(* Logix 5000 Rung export; software revision 17.00 *)

TYPE AENWG_CIP :   // Total Number of Current CIP Connections
STRUCT
   Opens : DINT;   // Total number of CIP connection Open Requests
   Closes : DINT;   // Total Number of CIP Connection Close Requests
   TimeOuts : DINT;   // Total Number of CIP Connection TimeOuts
END_STRUCT
END_TYPE

TYPE AENWG_PacketsRxSuccess :
STRUCT
   TotalCount : DINT;   // Total number of "good" received packets
   AvgPerSecond : DINT;   // Average "good" received packets per second
END_STRUCT
END_TYPE

TYPE AENWG_PacketsTxRetries :
STRUCT
   TotalCount : DINT;   // Total transmit packet retries
   AvgPerSecond : DINT;   // Average transmit packet retries per second
END_STRUCT
END_TYPE

TYPE AENWG_PacketsTxSuccess :
STRUCT
   TotalCount : DINT;   // Total "good" transmitted packets
   AvgPerSecond : DINT;   // Average "good" transmitted packets per second
END_STRUCT
END_TYPE

TYPE AENWG_PacketsTxFailures :
STRUCT
   TotalCount : DINT;   // Total number of failed transmitted packets
   AvgPerSecond : DINT;   // Average failed packets per second
END_STRUCT
END_TYPE

TYPE AENWG_RadioLinkTime :
STRUCT
   Days : INT;   // Number of days the radio has been linked to a parent
   Hours : INT;   // Number of hours the radio has been linked to a parent
   Minutes : INT;   // Number of minutes the radio has been linked to a parent
   Seconds : INT;   // Number of seconds the radio has been linked to a parent
END_STRUCT
END_TYPE

TYPE AENWG_DIAGNOSTICS :
STRUCT
   Control : AENWG_CONTROL;
   HMI : AENWG_HMI;
END_STRUCT
END_TYPE

TYPE AENWG_HMI :
STRUCT
   Face_Plate_Nav : DINT;   // Used by the HMI for display navigation
   RadioFirmware : DINT;   // Current radio firmware revision
   Module_Comm_Status : INT;
   ParentDataRate : INT;   // The data rate at which the parent is transmitting data *IN Mbps
   RSSI : INT;   // Current receive signal strength
   SignalToNoise : INT;   // Current noise level
   LinkTime : AENWG_RadioLinkTime;   // Total time the radio has been linked to a master
   ParentMACaddress : AENWG_ParentMACAddress;   // The MAC address of the linked parent
   TxPackets_Success : AENWG_PacketsTxSuccess;   // Total and average "good" packets
   TxPackets_Fail : AENWG_PacketsTxFailures;   // Total and average failed packets
   TxPackets_Retries : AENWG_PacketsTxRetries;   // Total and average retries
   RxPackets_Success : AENWG_PacketsRxSuccess;   // Total and average received packets
   IPInformation : AENWG_IPData;   // ILX34 TCP information
   CIP : AENWG_CIP;   // ILX34 CIP Connection Data
END_STRUCT
END_TYPE

TYPE AENWG_ParentMACAddress :
STRUCT
   Octet1 : SINT;   // Octet1 of the parent's MAC address
   Octet2 : SINT;   // Octet2 of the parent's MAC address
   Octet3 : SINT;   // Octet3 of the parent's MAC address
   Octet4 : SINT;   // Octet4 of the parent's MAC address
   Octet5 : SINT;   // Octet5 of the parent's MAC address
   Octet6 : SINT;   // Octet6 of the parent's MAC address
END_STRUCT
END_TYPE

TYPE AENWG_IPData :   // contains the IP information related to the ILX34.
STRUCT
   IPAddress : INT[4];
   NetworkSubMask : INT[4];
   GatewayAddress : INT[4];
   DNSServer : INT[4];
   DNSServer2 : INT[4];
   IP_Msg_Trigger : DINT;
END_STRUCT
END_TYPE

TYPE AENWG_CONTROL :
STRUCT
   ConMsgData : INT[12];   // Array that stores temporary connection data from the ILX34
   RadioMsgData : INT[36];   // Array that stores the temporary data from the ILX34
   IPMsgData : DINT[10];   // Array that stores temporary data for the IP information
   PollRate : DINT;   // Poll rate for retrieving radio diagnostic data *IN SECONDS
   RadioPollTimer : TIMER;   // Interval at which to get diagnostics from the ILX34 (should not be faster than every 3 sec)
END_STRUCT
END_TYPE

ADD_ON_INSTRUCTION ILX34AENWG_Advanced   (* revision 1.0, vendor ProSoft Technology, ExecutePrescan *)
// This is the Advanced Add On Instruction that provides the ability to get diagnostic information from an ILX34AENWG.
VAR_IN_OUT
   ILX34_Diag_msg : MESSAGE; {required}
   WirelessAENWG_Diags : AENWG_DIAGNOSTICS; {required}
   ILX34_IP_Info_msg : MESSAGE; {required}
   ILX34_Con_Diag_msg : MESSAGE; {required}
END_VAR
VAR
   Move_IP_Data : BOOL;
   IP_Domain_Name_Size : DINT;
   Move_Wireless_Diag : BOOL;
END_VAR

ROUTINE Logic   (* ladder *)
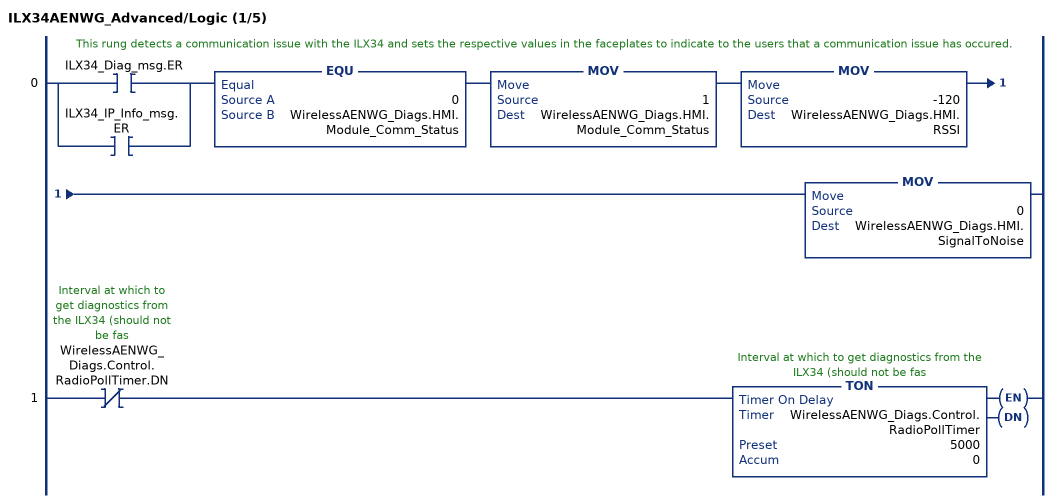
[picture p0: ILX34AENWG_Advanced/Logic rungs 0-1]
   // This rung detects a communication issue with the ILX34 and sets the respective values in the faceplates to indicate to the users that a communication issue has occured.
   0: [XIC(ILX34_Diag_msg.ER) ,XIC(ILX34_IP_Info_msg.ER) ]EQU(0,WirelessAENWG_Diags.HMI.Module_Comm_Status)MOV(1,WirelessAENWG_Diags.HMI.Module_Comm_Status)MOV(-120,WirelessAENWG_Diags.HMI.RSSI)MOV(0,WirelessAENWG_Diags.HMI.SignalToNoise);
   1: XIO(WirelessAENWG_Diags.Control.RadioPollTimer.DN)TON(WirelessAENWG_Diags.Control.RadioPollTimer,5000,0);
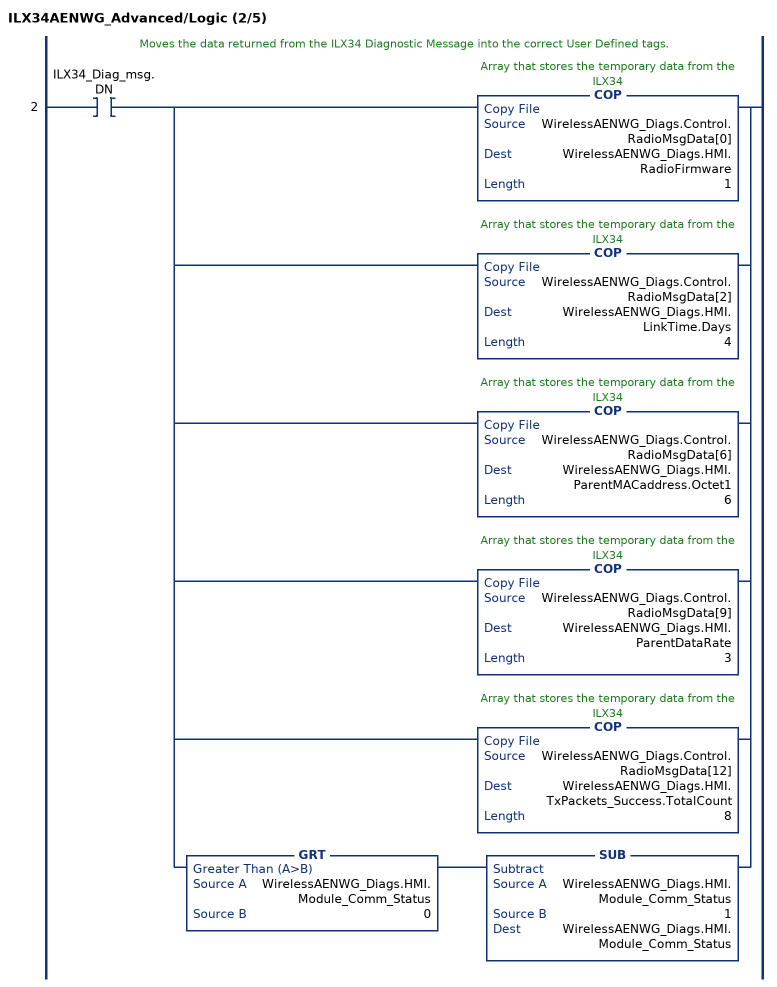
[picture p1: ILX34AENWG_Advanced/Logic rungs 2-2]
   // Moves the data returned from the ILX34 Diagnostic Message into the correct User Defined tags.
   2: XIC(ILX34_Diag_msg.DN)[COP(WirelessAENWG_Diags.Control.RadioMsgData[0],WirelessAENWG_Diags.HMI.RadioFirmware,1) ,COP(WirelessAENWG_Diags.Control.RadioMsgData[2],WirelessAENWG_Diags.HMI.LinkTime.Days,4) ,COP(WirelessAENWG_Diags.Control.RadioMsgData[6],WirelessAENWG_Diags.HMI.ParentMACaddress.Octet1,6) ,COP(WirelessAENWG_Diags.Control.RadioMsgData[9],WirelessAENWG_Diags.HMI.ParentDataRate,3) ,COP(WirelessAENWG_Diags.Control.RadioMsgData[12],WirelessAENWG_Diags.HMI.TxPackets_Success.TotalCount,8) ,GRT(WirelessAENWG_Diags.HMI.Module_Comm_Status,0) SUB(WirelessAENWG_Diags.HMI.Module_Comm_Status,1,WirelessAENWG_Diags.HMI.Module_Comm_Status) ];
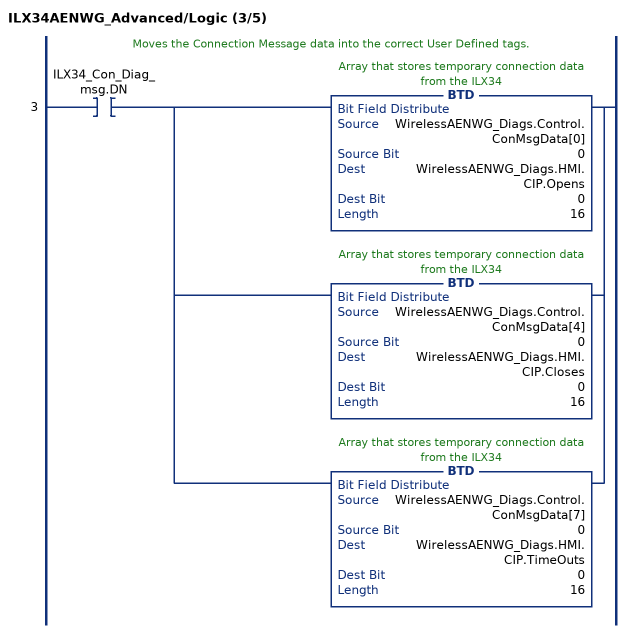
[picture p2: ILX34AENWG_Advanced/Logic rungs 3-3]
   // Moves the Connection Message data into the correct User Defined tags.
   3: XIC(ILX34_Con_Diag_msg.DN)[BTD(WirelessAENWG_Diags.Control.ConMsgData[0],0,WirelessAENWG_Diags.HMI.CIP.Opens,0,16) ,BTD(WirelessAENWG_Diags.Control.ConMsgData[4],0,WirelessAENWG_Diags.HMI.CIP.Closes,0,16) ,BTD(WirelessAENWG_Diags.Control.ConMsgData[7],0,WirelessAENWG_Diags.HMI.CIP.TimeOuts,0,16) ];
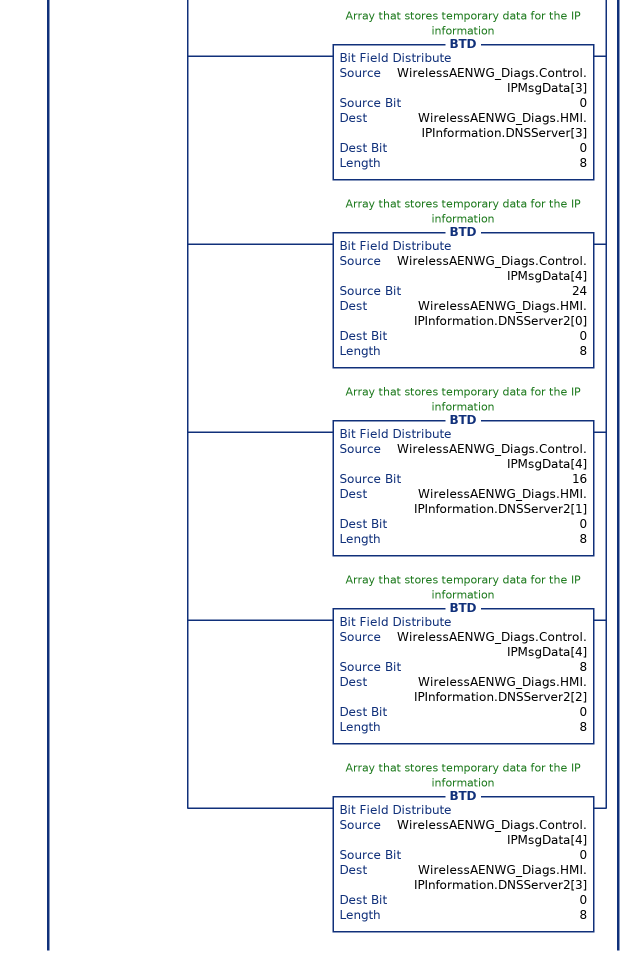
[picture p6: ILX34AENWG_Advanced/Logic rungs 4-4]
   // Moves the IP related information returned from the ILX34 IP msg into the correct user defined data types.
   4: XIC(ILX34_IP_Info_msg.DN)[[BTD(WirelessAENWG_Diags.Control.IPMsgData[0],24,WirelessAENWG_Diags.HMI.IPInformation.IPAddress[0],0,8) ,BTD(WirelessAENWG_Diags.Control.IPMsgData[0],16,WirelessAENWG_Diags.HMI.IPInformation.IPAddress[1],0,8) ,BTD(WirelessAENWG_Diags.Control.IPMsgData[0],8,WirelessAENWG_Diags.HMI.IPInformation.IPAddress[2],0,8) ,BTD(WirelessAENWG_Diags.Control.IPMsgData[0],0,WirelessAENWG_Diags.HMI.IPInformation.IPAddress[3],0,8) ] ,[BTD(WirelessAENWG_Diags.Control.IPMsgData[1],24,WirelessAENWG_Diags.HMI.IPInformation.NetworkSubMask[0],0,8) ,BTD(WirelessAENWG_Diags.Control.IPMsgData[1],16,WirelessAENWG_Diags.HMI.IPInformation.NetworkSubMask[1],0,8) ,BTD(WirelessAENWG_Diags.Control.IPMsgData[1],8,WirelessAENWG_Diags.HMI.IPInformation.NetworkSubMask[2],0,8) ,BTD(WirelessAENWG_Diags.Control.IPMsgData[1],0,WirelessAENWG_Diags.HMI.IPInformation.NetworkSubMask[3],0,8) ] ,[BTD(WirelessAENWG_Diags.Control.IPMsgData[2],24,WirelessAENWG_Diags.HMI.IPInformation.GatewayAddress[0],0,8) ,BTD(WirelessAENWG_Diags.Control.IPMsgData[2],16,WirelessAENWG_Diags.HMI.IPInformation.GatewayAddress[1],0,8) ,BTD(WirelessAENWG_Diags.Control.IPMsgData[2],8,WirelessAENWG_Diags.HMI.IPInformation.GatewayAddress[2],0,8) ,BTD(WirelessAENWG_Diags.Control.IPMsgData[2],0,WirelessAENWG_Diags.HMI.IPInformation.GatewayAddress[3],0,8) ] ,[BTD(WirelessAENWG_Diags.Control.IPMsgData[3],24,WirelessAENWG_Diags.HMI.IPInformation.DNSServer[0],0,8) ,BTD(WirelessAENWG_Diags.Control.IPMsgData[3],16,WirelessAENWG_Diags.HMI.IPInformation.DNSServer[1],0,8) ,BTD(WirelessAENWG_Diags.Control.IPMsgData[3],8,WirelessAENWG_Diags.HMI.IPInformation.DNSServer[2],0,8) ,BTD(WirelessAENWG_Diags.Control.IPMsgData[3],0,WirelessAENWG_Diags.HMI.IPInformation.DNSServer[3],0,8) ] ,[BTD(WirelessAENWG_Diags.Control.IPMsgData[4],24,WirelessAENWG_Diags.HMI.IPInformation.DNSServer2[0],0,8) ,BTD(WirelessAENWG_Diags.Control.IPMsgData[4],16,WirelessAENWG_Diags.HMI.IPInformation.DNSServer2[1],0,8) ,BTD(WirelessAENWG_Diags.Control.IPMsgData[4],8,WirelessAENWG_Diags.HMI.IPInformation.DNSServer2[2],0,8) ,BTD(WirelessAENWG_Diags.Control.IPMsgData[4],0,WirelessAENWG_Diags.HMI.IPInformation.DNSServer2[3],0,8) ] ];
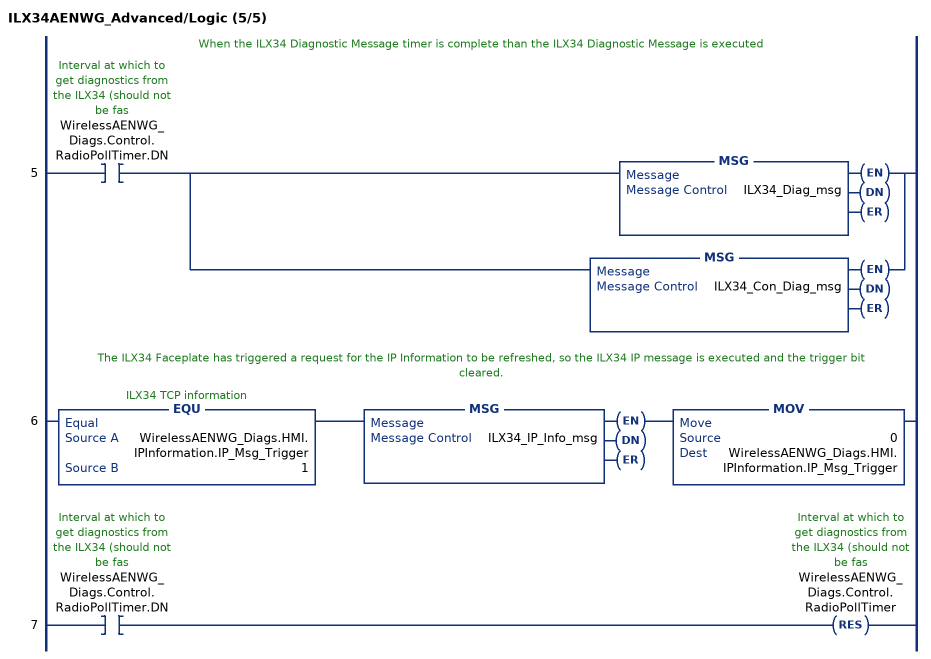
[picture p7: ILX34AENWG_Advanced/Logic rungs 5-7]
   // When the ILX34 Diagnostic Message timer is complete than the ILX34 Diagnostic Message is executed
   5: XIC(WirelessAENWG_Diags.Control.RadioPollTimer.DN)[MSG(ILX34_Diag_msg) ,MSG(ILX34_Con_Diag_msg) ];
   // The ILX34 Faceplate has triggered a request for the IP Information to be refreshed, so the ILX34 IP message is executed and the trigger bit cleared.
   6: EQU(WirelessAENWG_Diags.HMI.IPInformation.IP_Msg_Trigger,1)MSG(ILX34_IP_Info_msg)MOV(0,WirelessAENWG_Diags.HMI.IPInformation.IP_Msg_Trigger);
   7: XIC(WirelessAENWG_Diags.Control.RadioPollTimer.DN)RES(WirelessAENWG_Diags.Control.RadioPollTimer);
END_ROUTINE

ROUTINE Prescan   (* ladder *)
// Fire diagnostics messages in order to get initial data.
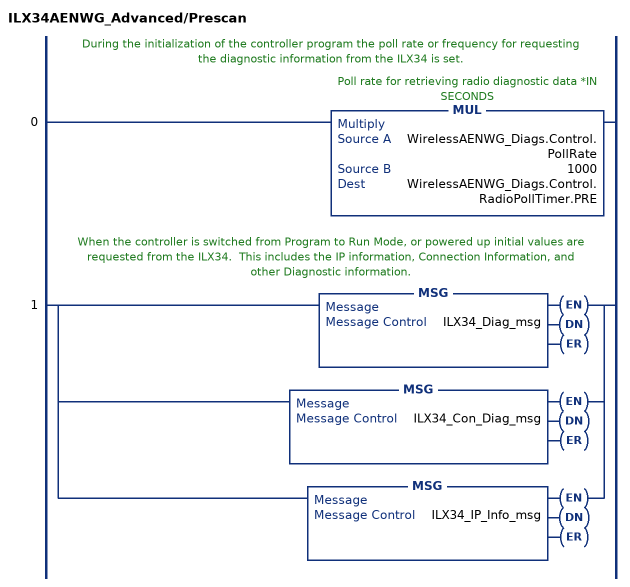
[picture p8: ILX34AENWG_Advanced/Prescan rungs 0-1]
   // During the initialization of the controller program the poll rate or frequency for requesting the diagnostic information from the ILX34 is set.
   0: MUL(WirelessAENWG_Diags.Control.PollRate,1000,WirelessAENWG_Diags.Control.RadioPollTimer.PRE);
   // When the controller is switched from Program to Run Mode, or powered up initial values are requested from the ILX34.  This includes the IP information, Connection Information, and other Diagnostic information.
   1: [MSG(ILX34_Diag_msg) ,MSG(ILX34_Con_Diag_msg) ,MSG(ILX34_IP_Info_msg) ];
END_ROUTINE
END_ADD_ON_INSTRUCTION

VAR_GLOBAL   (* controller tags *)
   AENWG_Addon : ILX34AENWG_Advanced;
   ILX34_AENWG_Con_Msg : MESSAGE;
        MessageParameters(MessageType := CIP Generic, RequestedLength := 1, ConnectedFlag := 2, ConnectionPath := Enet, 2, 10.1.2.79, ServiceCode := 16#0001, ObjectType := 16#0006, TargetObject := 1, LocalElement := ILX34_AENWG.Control.ConMsgData[0], DestinationTag := ILX34_AENWG.Control.ConMsgData[0])
   ILX34_AENWG_Diag_Msg : MESSAGE;
        MessageParameters(MessageType := CIP Generic, RequestedLength := 1, ConnectedFlag := 2, ConnectionPath := Enet, 2, 10.1.2.79, ServiceCode := 16#0001, ObjectType := 16#0065, TargetObject := 1, LocalElement := ILX34_AENWG.Control.RadioMsgData[0], DestinationTag := ILX34_AENWG.Control.RadioMsgData[0])
   ILX34_AENWG : AENWG_DIAGNOSTICS := (Control.RadioPollTimer.PRE := 4000, ...);
   ILX34_AENWG_IP_Info_Msg : MESSAGE;
        MessageParameters(MessageType := CIP Generic, ConnectedFlag := 2, ConnectionPath := Enet, 2, 10.1.2.79, ServiceCode := 16#000e, ObjectType := 16#00f5, TargetObject := 1, AttributeNumber := 16#0005, DestinationTag := ILX34_AENWG.Control.IPMsgData[0])
END_VAR

PROGRAM Diagnostics

ROUTINE ILX34   (* ladder *)
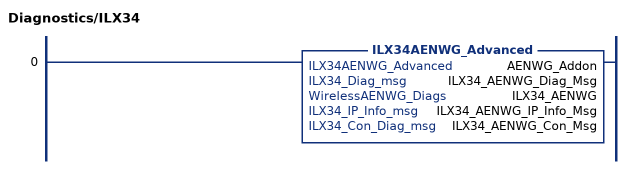
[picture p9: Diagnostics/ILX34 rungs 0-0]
   0: ILX34AENWG_Advanced(AENWG_Addon,ILX34_AENWG_Diag_Msg,ILX34_AENWG,ILX34_AENWG_IP_Info_Msg,ILX34_AENWG_Con_Msg);
END_ROUTINE
END_PROGRAM
